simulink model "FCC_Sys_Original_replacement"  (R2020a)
settings: Solver=FixedStepDiscrete  StartTime=0.0  StopTime=10.0  FixedStep=0.001  RelTol=1e-3  EnableMultiTasking=on
model workspace (MAT data in the model file):
  Ts : Simulink.Parameter (value not decoded)
  carriedVarFromRefMdlDV_0_Ts = 0.01
symbols that are objects in the model workspace (value not decoded): Ts
undefined symbols (not defined in the file or in its folder): ActuatorLoop, AHRS_voter, DiscIntNeverNeededParam, FCC, Heli_inner_loop, Heli_outer_loop, Kd, Ki, Kp, Normal
libraries: simulink x10, HeliLibrary x3

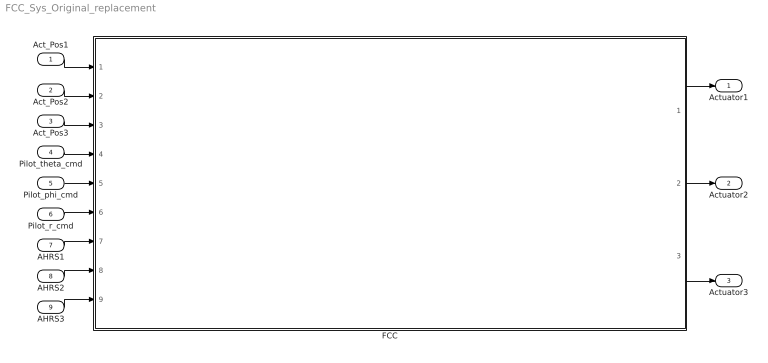
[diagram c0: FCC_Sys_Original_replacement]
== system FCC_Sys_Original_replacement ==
  Act_Pos1 : Inport  OutMin=-32768  OutMax=32767  OutDataTypeStr=int16  PortDimensions=1  SampleTime=0.001
  Act_Pos2 : Inport  Port=2  OutMin=-32768  OutMax=32767  OutDataTypeStr=int16  PortDimensions=1  SampleTime=0.001
  Act_Pos3 : Inport  Port=3  OutMin=-32768  OutMax=32767  OutDataTypeStr=int16  PortDimensions=1  SampleTime=0.001
  Pilot_theta_cmd : Inport  Port=4  OutMin=-32768  OutMax=32767  OutDataTypeStr=int16  PortDimensions=1  SampleTime=0.01
  Pilot_phi_cmd : Inport  Port=5  OutMin=-32768  OutMax=32767  OutDataTypeStr=int16  PortDimensions=1  SampleTime=0.01
  Pilot_r_cmd : Inport  Port=6  OutMin=-32768  OutMax=32767  OutDataTypeStr=int16  PortDimensions=1  SampleTime=0.01
  AHRS1 : Inport  Port=7  OutDataTypeStr=Bus: AHRS_Bus  PortDimensions=1  SampleTime=0.01
  AHRS2 : Inport  Port=8  OutDataTypeStr=Bus: AHRS_Bus  PortDimensions=1  SampleTime=0.01
  AHRS3 : Inport  Port=9  OutDataTypeStr=Bus: AHRS_Bus  PortDimensions=1  SampleTime=0.01
  FCC : Subsystem  TreatAsAtomicUnit=on  mask(Sldv ModelReference(Model name:FCC) Replacement){ModelName=FCC, ParameterArgumentNames=, ParameterArgumentValuesAsString=, SimulationMode=Normal}
      mask help: Replacement for the Model Reference block that references the model FCC. If Model arguments are specified on the Model Reference block, then they will appear in the mask parameters.
  Actuator1 : Outport  VectorParamsAs1DForOutWhenUnconnected=off
  Actuator2 : Outport  Port=2  VectorParamsAs1DForOutWhenUnconnected=off
  Actuator3 : Outport  Port=3  VectorParamsAs1DForOutWhenUnconnected=off
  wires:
  Act_Pos1/1 -> FCC/1(Act_Pos1)
  Act_Pos2/1 -> FCC/2(Act_Pos2)
  Act_Pos3/1 -> FCC/3(Act_Pos3)
  Pilot_theta_cmd/1 -> FCC/4(Pilot_theta_cmd)
  Pilot_phi_cmd/1 -> FCC/5(Pilot_phi_cmd)
  Pilot_r_cmd/1 -> FCC/6(Pilot_r_cmd)
  AHRS1/1 -> FCC/7(AHRS1)
  AHRS2/1 -> FCC/8(AHRS2)
  AHRS3/1 -> FCC/9(AHRS3)
  FCC/1(Actuator1) -> Actuator1/1
  FCC/2(Actuator2) -> Actuator2/1
  FCC/3(Actuator3) -> Actuator3/1

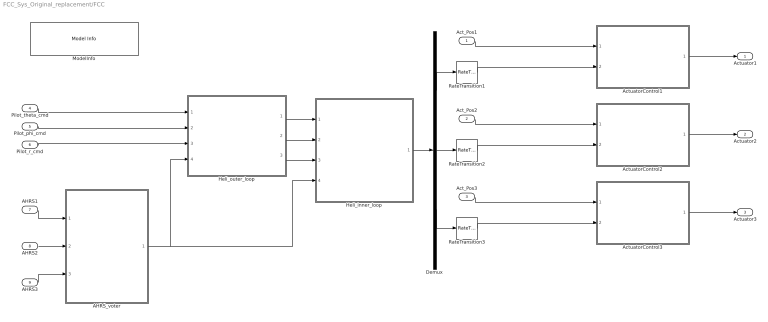
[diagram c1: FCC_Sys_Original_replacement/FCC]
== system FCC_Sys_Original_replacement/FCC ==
  Act_Pos1 : Inport  OutMin=-32768  OutMax=32767  OutDataTypeStr=int16  PortDimensions=1  SampleTime=[0.001,0]
  Act_Pos2 : Inport  Port=2  OutMin=-32768  OutMax=32767  OutDataTypeStr=int16  PortDimensions=1  SampleTime=[0.001,0]
  Act_Pos3 : Inport  Port=3  OutMin=-32768  OutMax=32767  OutDataTypeStr=int16  PortDimensions=1  SampleTime=[0.001,0]
  Pilot_theta_cmd : Inport  Port=4  OutMin=-32768  OutMax=32767  OutDataTypeStr=int16  PortDimensions=1  SampleTime=[0.01,0]
  Pilot_phi_cmd : Inport  Port=5  OutMin=-32768  OutMax=32767  OutDataTypeStr=int16  PortDimensions=1  SampleTime=[0.01,0]
  Pilot_r_cmd : Inport  Port=6  OutMin=-32768  OutMax=32767  OutDataTypeStr=int16  PortDimensions=1  SampleTime=[0.01,0]
  AHRS1 : Inport  Port=7  OutDataTypeStr=Bus: AHRS_Bus  PortDimensions=1  SampleTime=[0.01,0]
  AHRS2 : Inport  Port=8  OutDataTypeStr=Bus: AHRS_Bus  PortDimensions=1  SampleTime=[0.01,0]
  AHRS3 : Inport  Port=9  OutDataTypeStr=Bus: AHRS_Bus  PortDimensions=1  SampleTime=[0.01,0]
  AHRS_voter : Subsystem  TreatAsAtomicUnit=on  mask(Sldv ModelReference(Model name:AHRS_voter) Replacement){ModelName=AHRS_voter, ParameterArgumentNames=, ParameterArgumentValuesAsString=, SimulationMode=Normal}
      mask help: Replacement for the Model Reference block that references the model AHRS_voter. If Model arguments are specified on the Model Reference block, then they will appear in the mask parameters.
  ActuatorControl1 : Subsystem  TreatAsAtomicUnit=on  mask(Sldv ModelReference(Model name:ActuatorLoop) Replacement){Kd=double(0.00272), Ki=double(2.73), Kp=double(0.339), ModelName=ActuatorLoop, ParameterArgumentNames=Kd,Ki,Kp, ParameterArgumentValuesAsString=0.00272,2.73,0.339, SimulationMode=Normal}
      mask help: Replacement for the Model Reference block that references the model ActuatorLoop. If Model arguments are specified on the Model Reference block, then they will appear in the mask parameters.
  ActuatorControl2 : Subsystem  TreatAsAtomicUnit=on  mask(Sldv ModelReference(Model name:ActuatorLoop) Replacement){Kd=double(0.00272), Ki=double(2.73), Kp=double(0.339), ModelName=ActuatorLoop, ParameterArgumentNames=Kd,Ki,Kp, ParameterArgumentValuesAsString=0.00272,2.73,0.339, SimulationMode=Normal}
      mask help: Replacement for the Model Reference block that references the model ActuatorLoop. If Model arguments are specified on the Model Reference block, then they will appear in the mask parameters.
  ActuatorControl3 : Subsystem  TreatAsAtomicUnit=on  mask(Sldv ModelReference(Model name:ActuatorLoop) Replacement){Kd=double(0.00272), Ki=double(2.73), Kp=double(0.339), ModelName=ActuatorLoop, ParameterArgumentNames=Kd,Ki,Kp, ParameterArgumentValuesAsString=0.00272,2.73,0.339, SimulationMode=Normal}
      mask help: Replacement for the Model Reference block that references the model ActuatorLoop. If Model arguments are specified on the Model Reference block, then they will appear in the mask parameters.
  Demux : Demux  Outputs=3
  Heli_inner_loop : Subsystem  TreatAsAtomicUnit=on  mask(Sldv ModelReference(Model name:Heli_inner_loop) Replacement){ModelName=Heli_inner_loop, ParameterArgumentNames=, ParameterArgumentValuesAsString=, SimulationMode=Normal}
      mask help: Replacement for the Model Reference block that references the model Heli_inner_loop. If Model arguments are specified on the Model Reference block, then they will appear in the mask parameters.
  Heli_outer_loop : Subsystem  TreatAsAtomicUnit=on  mask(Sldv ModelReference(Model name:Heli_outer_loop) Replacement){Ts=carriedVarFromRefMdlDV_0_Ts, ModelName=Heli_outer_loop, ParameterArgumentNames=, ParameterArgumentValuesAsString=, SimulationMode=Normal}
      mask help: Replacement for the Model Reference block that references the model Heli_outer_loop. If Model arguments are specified on the Model Reference block, then they will appear in the mask parameters.
  ModelInfo : simulink/Model-Wide Utilities/Model Info  Frame=on  DisplayStringWithTags=|  HorizontalTextAlignment=Center  LeftAlignmentValue=0.5
      | Model Name: %<ModelName>
      | Model Version: %<ModelVersion>
      | Last Modified: %<LastModificationDate>
      | 
      | Copyright 2016 The MathWorks, Inc.
  RateTransition1 : RateTransition  OutPortSampleTime=0.001
  RateTransition2 : RateTransition  OutPortSampleTime=0.001
  RateTransition3 : RateTransition  OutPortSampleTime=0.001
  Actuator1 : Outport  OutDataTypeStr=int16  PortDimensions=1  SampleTime=[0.001,0]  VectorParamsAs1DForOutWhenUnconnected=off
  Actuator2 : Outport  Port=2  OutDataTypeStr=int16  PortDimensions=1  SampleTime=[0.001,0]  VectorParamsAs1DForOutWhenUnconnected=off
  Actuator3 : Outport  Port=3  OutDataTypeStr=int16  PortDimensions=1  SampleTime=[0.001,0]  VectorParamsAs1DForOutWhenUnconnected=off
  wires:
  AHRS_voter/1(voted_fb) -> Heli_inner_loop/4(voted_fb), Heli_outer_loop/4(voted_fb)
  ActuatorControl3/1(ActuatorCommand) -> Actuator3/1
  ActuatorControl2/1(ActuatorCommand) -> Actuator2/1
  ActuatorControl1/1(ActuatorCommand) -> Actuator1/1
  Act_Pos3/1 -> ActuatorControl3/1(PositionFeedback)
  Act_Pos2/1 -> ActuatorControl2/1(PositionFeedback)
  Act_Pos1/1 -> ActuatorControl1/1(PositionFeedback)
  Pilot_r_cmd/1 -> Heli_outer_loop/3(Pilot_r_cmd)
  Pilot_phi_cmd/1 -> Heli_outer_loop/2(Pilot_phi_cmd)
  Pilot_theta_cmd/1 -> Heli_outer_loop/1(Pilot_theta_cmd)
  AHRS1/1 -> AHRS_voter/1(AHRS1)
  Heli_outer_loop/3(r_cmd) -> Heli_inner_loop/3(r_cmd)
  Heli_outer_loop/2(phi_cmd) -> Heli_inner_loop/2(phi_cmd)
  Heli_outer_loop/1(theta_cmd) -> Heli_inner_loop/1(theta_cmd)
  Heli_inner_loop/1(actuator_commands) -> Demux/1
  Demux/3 -> RateTransition3/1
  Demux/2 -> RateTransition2/1
  Demux/1 -> RateTransition1/1
  AHRS3/1 -> AHRS_voter/3(AHRS3)
  AHRS2/1 -> AHRS_voter/2(AHRS2)
  RateTransition3/1 -> ActuatorControl3/2(PositionCommand)
  RateTransition2/1 -> ActuatorControl2/2(PositionCommand)
  RateTransition1/1 -> ActuatorControl1/2(PositionCommand)

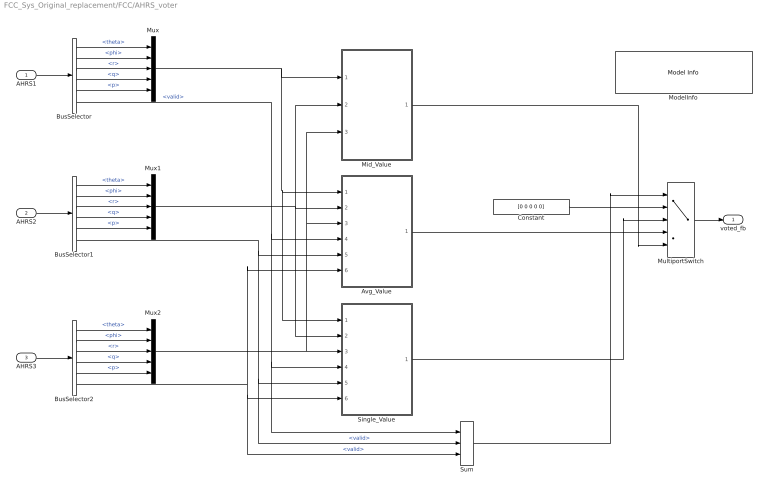
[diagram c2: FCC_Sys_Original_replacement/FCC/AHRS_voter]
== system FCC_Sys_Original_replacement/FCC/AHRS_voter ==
  AHRS1 : Inport  OutDataTypeStr=Bus: AHRS_Bus  PortDimensions=1  SampleTime=[0.01,0]
  AHRS2 : Inport  Port=2  OutDataTypeStr=Bus: AHRS_Bus  PortDimensions=1  SampleTime=[0.01,0]
  AHRS3 : Inport  Port=3  OutDataTypeStr=Bus: AHRS_Bus  PortDimensions=1  SampleTime=[0.01,0]
  Avg_Value : Subsystem  TreatAsAtomicUnit=on  RTWFcnName=Avg_Value
  BusSelector : BusSelector  OutputSignals=theta,phi,r,q,p,valid
  BusSelector1 : BusSelector  OutputSignals=theta,phi,r,q,p,valid
  BusSelector2 : BusSelector  OutputSignals=theta,phi,r,q,p,valid
  Constant : Constant  Value=[0 0 0 0 0]
  Mid_Value : Subsystem  TreatAsAtomicUnit=on  RTWFcnName=Mid_Value
  ModelInfo : simulink/Model-Wide Utilities/Model Info  Frame=on  DisplayStringWithTags=|  HorizontalTextAlignment=Center  LeftAlignmentValue=0.5
      | Model Name: %<ModelName>
      | Model Version: %<ModelVersion>
      | Last Modified: %<LastModificationDate>
      | 
      | Copyright 2016 The MathWorks, Inc.
  MultiportSwitch : MultiPortSwitch  DataPortOrder=Zero-based contiguous  Inputs=4  DiagnosticForDefault=None  zeroidx=on
  Mux : Mux  Inputs=5
  Mux1 : Mux  Inputs=5
  Mux2 : Mux  Inputs=5
  Single_Value : Subsystem  TreatAsAtomicUnit=on  RTWFcnName=Single_Value
  Sum : Sum  Inputs=+++  OutDataTypeStr=uint32
  voted_fb : Outport  OutDataTypeStr=double  PortDimensions=5  SampleTime=[0.01,0]  VectorParamsAs1DForOutWhenUnconnected=off
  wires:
  BusSelector2/6 -> Single_Value/6(AHRS3_Valid), Sum/3, Avg_Value/6(AHRS3_Valid)  "<valid>"
  BusSelector2/5 -> Mux2/5  "<p>"
  BusSelector2/4 -> Mux2/4  "<q>"
  BusSelector2/3 -> Mux2/3  "<r>"
  BusSelector2/2 -> Mux2/2  "<phi>"
  BusSelector2/1 -> Mux2/1  "<theta>"
  AHRS3/1 -> BusSelector2/1
  Mux2/1 -> Mid_Value/3(AHRS3), Avg_Value/3(AHRS3), Single_Value/3(AHRS3)
  BusSelector1/6 -> Avg_Value/5(AHRS2_Valid), Sum/2, Single_Value/5(AHRS2_Valid)  "<valid>"
  Mux1/1 -> Single_Value/2(AHRS2), Mid_Value/2(AHRS2), Avg_Value/2(AHRS2)
  AHRS2/1 -> BusSelector1/1
  BusSelector1/1 -> Mux1/1  "<theta>"
  BusSelector1/2 -> Mux1/2  "<phi>"
  BusSelector1/3 -> Mux1/3  "<r>"
  BusSelector1/4 -> Mux1/4  "<q>"
  BusSelector1/5 -> Mux1/5  "<p>"
  Mux/1 -> Single_Value/1(AHRS1), Avg_Value/1(AHRS1), Mid_Value/1(AHRS1)
  BusSelector/5 -> Mux/5  "<p>"
  BusSelector/4 -> Mux/4  "<q>"
  BusSelector/3 -> Mux/3  "<r>"
  BusSelector/2 -> Mux/2  "<phi>"
  BusSelector/1 -> Mux/1  "<theta>"
  BusSelector/6 -> Single_Value/4(AHRS1_Valid), Sum/1, Avg_Value/4(AHRS1_Valid)  "<valid>"
  AHRS1/1 -> BusSelector/1
  Constant/1 -> MultiportSwitch/2
  Single_Value/1(Single_Value) -> MultiportSwitch/3
  Avg_Value/1(Avg_Value) -> MultiportSwitch/4
  Mid_Value/1(Mid_Value) -> MultiportSwitch/5
  Sum/1 -> MultiportSwitch/1
  MultiportSwitch/1 -> voted_fb/1

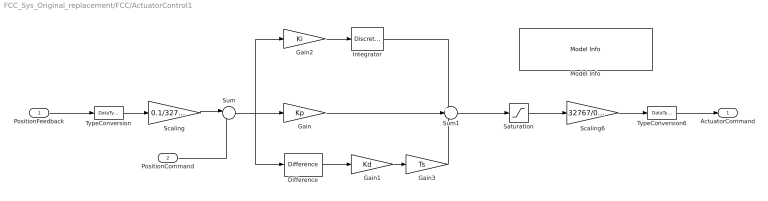
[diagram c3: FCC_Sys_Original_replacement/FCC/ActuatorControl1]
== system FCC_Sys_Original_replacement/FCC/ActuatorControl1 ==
  PositionFeedback : Inport  OutMin=-32768  OutMax=32767  OutDataTypeStr=int16  PortDimensions=1  SampleTime=[0.001,0]
  PositionCommand : Inport  Port=2  OutMin=-0.1  OutMax=0.1  OutDataTypeStr=double  PortDimensions=1  SampleTime=[0.001,0]
  Difference : simulink/Discrete/Difference  ICPrevInput=0.0  OutMin=[]  OutMax=[]  OutDataType=fixdt(1, 16)  OutScaling=2^-10  DoSatur=off
  Gain : Gain  Gain=Kp
  Gain1 : Gain  Gain=Kd
  Gain2 : Gain  Gain=Ki
  Gain3 : Gain  Gain=Ts
  Integrator : DiscreteIntegrator  SampleTime=-1  LimitOutput=on  UpperSaturationLimit=0.1  LowerSaturationLimit=-0.1  ICPrevOutput=DiscIntNeverNeededParam  ICPrevScaledInput=DiscIntNeverNeededParam
  Model Info : simulink/Model-Wide Utilities/Model Info  Frame=on  DisplayStringWithTags=|  HorizontalTextAlignment=Center  LeftAlignmentValue=0.5
      | Model Name: %<ModelName>
      | Model Version: %<ModelVersion>
      | Last Modified: %<LastModificationDate>
      | 
      | Copyright 2016 The MathWorks, Inc.
  Saturation : Saturate  UpperLimit=0.3  LowerLimit=-0.3
  Scaling : Gain  Gain=0.1/32767
  Scaling6 : Gain  Gain=32767/0.3  SaturateOnIntegerOverflow=on
  Sum : Sum  Inputs=|-+
  Sum1 : Sum  Inputs=++-
  TypeConversion : DataTypeConversion  OutDataTypeStr=double
  TypeConversion6 : DataTypeConversion  OutDataTypeStr=int16
  ActuatorCommand : Outport  OutDataTypeStr=int16  PortDimensions=1  SampleTime=[0.001,0]  VectorParamsAs1DForOutWhenUnconnected=off
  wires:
  Gain3/1 -> Sum1/3
  TypeConversion6/1 -> ActuatorCommand/1
  Saturation/1 -> Scaling6/1
  Scaling6/1 -> TypeConversion6/1
  Scaling/1 -> Sum/1
  TypeConversion/1 -> Scaling/1
  PositionFeedback/1 -> TypeConversion/1
  Gain2/1 -> Integrator/1
  Gain1/1 -> Gain3/1
  Difference/1 -> Gain1/1
  Integrator/1 -> Sum1/1
  Sum1/1 -> Saturation/1
  Gain/1 -> Sum1/2
  Sum/1 -> Difference/1, Gain2/1, Gain/1
  PositionCommand/1 -> Sum/2

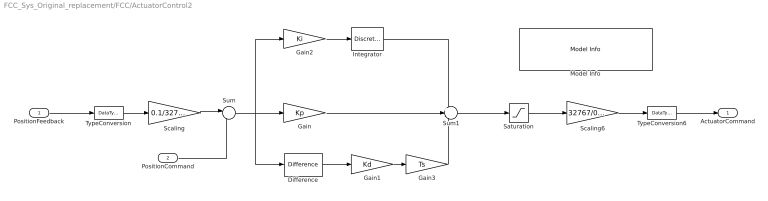
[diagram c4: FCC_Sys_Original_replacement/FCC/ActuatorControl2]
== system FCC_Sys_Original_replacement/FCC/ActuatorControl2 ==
  PositionFeedback : Inport  OutMin=-32768  OutMax=32767  OutDataTypeStr=int16  PortDimensions=1  SampleTime=[0.001,0]
  PositionCommand : Inport  Port=2  OutMin=-0.1  OutMax=0.1  OutDataTypeStr=double  PortDimensions=1  SampleTime=[0.001,0]
  Difference : simulink/Discrete/Difference  ICPrevInput=0.0  OutMin=[]  OutMax=[]  OutDataType=fixdt(1, 16)  OutScaling=2^-10  DoSatur=off
  Gain : Gain  Gain=Kp
  Gain1 : Gain  Gain=Kd
  Gain2 : Gain  Gain=Ki
  Gain3 : Gain  Gain=Ts
  Integrator : DiscreteIntegrator  SampleTime=-1  LimitOutput=on  UpperSaturationLimit=0.1  LowerSaturationLimit=-0.1  ICPrevOutput=DiscIntNeverNeededParam  ICPrevScaledInput=DiscIntNeverNeededParam
  Model Info : simulink/Model-Wide Utilities/Model Info  Frame=on  DisplayStringWithTags=|  HorizontalTextAlignment=Center  LeftAlignmentValue=0.5
      | Model Name: %<ModelName>
      | Model Version: %<ModelVersion>
      | Last Modified: %<LastModificationDate>
      | 
      | Copyright 2016 The MathWorks, Inc.
  Saturation : Saturate  UpperLimit=0.3  LowerLimit=-0.3
  Scaling : Gain  Gain=0.1/32767
  Scaling6 : Gain  Gain=32767/0.3  SaturateOnIntegerOverflow=on
  Sum : Sum  Inputs=|-+
  Sum1 : Sum  Inputs=++-
  TypeConversion : DataTypeConversion  OutDataTypeStr=double
  TypeConversion6 : DataTypeConversion  OutDataTypeStr=int16
  ActuatorCommand : Outport  OutDataTypeStr=int16  PortDimensions=1  SampleTime=[0.001,0]  VectorParamsAs1DForOutWhenUnconnected=off
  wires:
  Gain3/1 -> Sum1/3
  TypeConversion6/1 -> ActuatorCommand/1
  Saturation/1 -> Scaling6/1
  Scaling6/1 -> TypeConversion6/1
  Scaling/1 -> Sum/1
  TypeConversion/1 -> Scaling/1
  PositionFeedback/1 -> TypeConversion/1
  Gain2/1 -> Integrator/1
  Gain1/1 -> Gain3/1
  Difference/1 -> Gain1/1
  Integrator/1 -> Sum1/1
  Sum1/1 -> Saturation/1
  Gain/1 -> Sum1/2
  Sum/1 -> Difference/1, Gain2/1, Gain/1
  PositionCommand/1 -> Sum/2

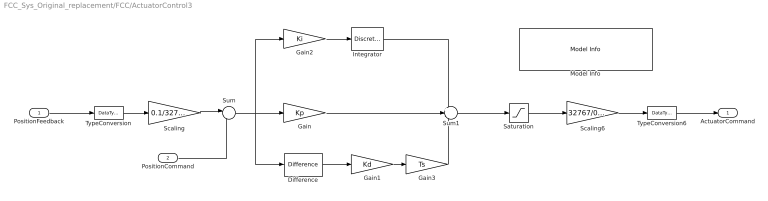
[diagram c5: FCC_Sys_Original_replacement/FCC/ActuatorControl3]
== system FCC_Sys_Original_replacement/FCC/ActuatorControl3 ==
  PositionFeedback : Inport  OutMin=-32768  OutMax=32767  OutDataTypeStr=int16  PortDimensions=1  SampleTime=[0.001,0]
  PositionCommand : Inport  Port=2  OutMin=-0.1  OutMax=0.1  OutDataTypeStr=double  PortDimensions=1  SampleTime=[0.001,0]
  Difference : simulink/Discrete/Difference  ICPrevInput=0.0  OutMin=[]  OutMax=[]  OutDataType=fixdt(1, 16)  OutScaling=2^-10  DoSatur=off
  Gain : Gain  Gain=Kp
  Gain1 : Gain  Gain=Kd
  Gain2 : Gain  Gain=Ki
  Gain3 : Gain  Gain=Ts
  Integrator : DiscreteIntegrator  SampleTime=-1  LimitOutput=on  UpperSaturationLimit=0.1  LowerSaturationLimit=-0.1  ICPrevOutput=DiscIntNeverNeededParam  ICPrevScaledInput=DiscIntNeverNeededParam
  Model Info : simulink/Model-Wide Utilities/Model Info  Frame=on  DisplayStringWithTags=|  HorizontalTextAlignment=Center  LeftAlignmentValue=0.5
      | Model Name: %<ModelName>
      | Model Version: %<ModelVersion>
      | Last Modified: %<LastModificationDate>
      | 
      | Copyright 2016 The MathWorks, Inc.
  Saturation : Saturate  UpperLimit=0.3  LowerLimit=-0.3
  Scaling : Gain  Gain=0.1/32767
  Scaling6 : Gain  Gain=32767/0.3  SaturateOnIntegerOverflow=on
  Sum : Sum  Inputs=|-+
  Sum1 : Sum  Inputs=++-
  TypeConversion : DataTypeConversion  OutDataTypeStr=double
  TypeConversion6 : DataTypeConversion  OutDataTypeStr=int16
  ActuatorCommand : Outport  OutDataTypeStr=int16  PortDimensions=1  SampleTime=[0.001,0]  VectorParamsAs1DForOutWhenUnconnected=off
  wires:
  Gain3/1 -> Sum1/3
  TypeConversion6/1 -> ActuatorCommand/1
  Saturation/1 -> Scaling6/1
  Scaling6/1 -> TypeConversion6/1
  Scaling/1 -> Sum/1
  TypeConversion/1 -> Scaling/1
  PositionFeedback/1 -> TypeConversion/1
  Gain2/1 -> Integrator/1
  Gain1/1 -> Gain3/1
  Difference/1 -> Gain1/1
  Integrator/1 -> Sum1/1
  Sum1/1 -> Saturation/1
  Gain/1 -> Sum1/2
  Sum/1 -> Difference/1, Gain2/1, Gain/1
  PositionCommand/1 -> Sum/2

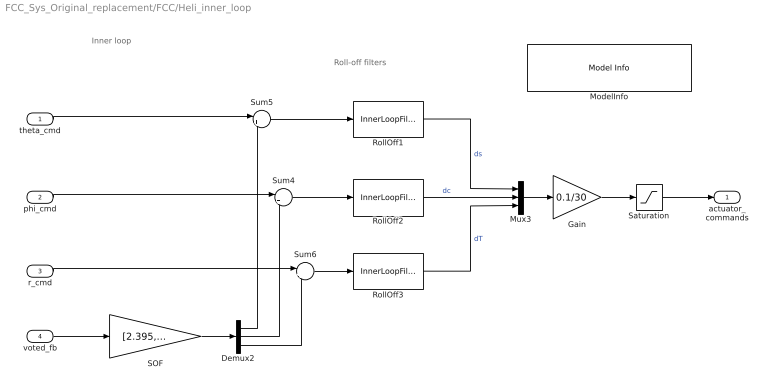
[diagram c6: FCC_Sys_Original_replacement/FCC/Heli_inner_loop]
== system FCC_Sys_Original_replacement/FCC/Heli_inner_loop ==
  note: Inner loop
  note: Roll-off filters
  theta_cmd : Inport  OutMin=-30  OutMax=30  OutDataTypeStr=double  PortDimensions=1  SampleTime=[0.01,0]
  phi_cmd : Inport  Port=2  OutMin=-30  OutMax=30  OutDataTypeStr=double  PortDimensions=1  SampleTime=[0.01,0]
  r_cmd : Inport  Port=3  OutMin=-30  OutMax=30  OutDataTypeStr=double  PortDimensions=1  SampleTime=[0.01,0]
  voted_fb : Inport  Port=4  OutMin=-180  OutMax=180  OutDataTypeStr=double  PortDimensions=5  SampleTime=[0.01,0]
  Demux2 : Demux  Outputs=3
  Gain : Gain  Gain=0.1/30
  ModelInfo : simulink/Model-Wide Utilities/Model Info  Frame=on  DisplayStringWithTags=|  HorizontalTextAlignment=Center  LeftAlignmentValue=0.5
      | Model Name: %<ModelName>
      | Model Version: %<ModelVersion>
      | Last Modified: %<LastModificationDate>
      | 
      | Copyright 2016 The MathWorks, Inc.
  Mux3 : Mux  Inputs=3
  RollOff1 : HeliLibrary/InnerLoopFilter  Tag=FilterWizardSubSystem  SystemSampleTime=-1  Latency=0  AutoFrameSizeCalculation=off
  RollOff2 : HeliLibrary/InnerLoopFilter  Tag=FilterWizardSubSystem  SystemSampleTime=-1  Latency=0  AutoFrameSizeCalculation=off
  RollOff3 : HeliLibrary/InnerLoopFilter  Tag=FilterWizardSubSystem  SystemSampleTime=-1  Latency=0  AutoFrameSizeCalculation=off
  SOF : Gain  Gain=[2.395, -0.3609, -0.002145, 0.8087, -0.0205; -0.1427, -1.115, 0.04573, -0.04318, -0.1007; -0.02792, -0.02229, -2.025, -0.06152, 0.03151;]  Multiplication=Matrix(K*u) (u vector)
  Saturation : Saturate  UpperLimit=0.1  LowerLimit=-0.1
  Sum4 : Sum  Inputs=|+-
  Sum5 : Sum  Inputs=|+-
  Sum6 : Sum  Inputs=|+-
  actuator_commands : Outport  OutDataTypeStr=double  PortDimensions=3  SampleTime=[0.01,0]  VectorParamsAs1DForOutWhenUnconnected=off
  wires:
  Saturation/1 -> actuator_commands/1
  Gain/1 -> Saturation/1
  voted_fb/1 -> SOF/1
  Demux2/3 -> Sum6/2
  Demux2/2 -> Sum4/2
  Demux2/1 -> Sum5/2
  Sum6/1 -> RollOff3/1
  r_cmd/1 -> Sum6/1
  phi_cmd/1 -> Sum4/1
  SOF/1 -> Demux2/1
  Sum5/1 -> RollOff1/1
  theta_cmd/1 -> Sum5/1
  RollOff1/1 -> Mux3/1  "ds"
  RollOff2/1 -> Mux3/2  "dc"
  RollOff3/1 -> Mux3/3  "dT"
  Sum4/1 -> RollOff2/1
  Mux3/1 -> Gain/1

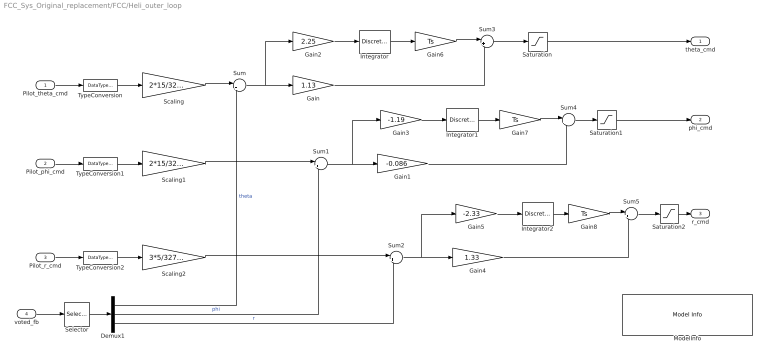
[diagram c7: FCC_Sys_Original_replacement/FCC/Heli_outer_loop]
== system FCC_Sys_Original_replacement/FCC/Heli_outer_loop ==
  Pilot_theta_cmd : Inport  OutMin=-32768  OutMax=32767  OutDataTypeStr=int16  PortDimensions=1  SampleTime=[0.01,0]
  Pilot_phi_cmd : Inport  Port=2  OutMin=-32768  OutMax=32767  OutDataTypeStr=int16  PortDimensions=1  SampleTime=[0.01,0]
  Pilot_r_cmd : Inport  Port=3  OutMin=-32768  OutMax=32767  OutDataTypeStr=int16  PortDimensions=1  SampleTime=[0.01,0]
  voted_fb : Inport  Port=4  OutMin=-180  OutMax=180  OutDataTypeStr=double  PortDimensions=5  SampleTime=[0.01,0]
  Demux1 : Demux  Outputs=3
  Gain : Gain  Gain=1.13
  Gain1 : Gain  Gain=-0.086
  Gain2 : Gain  Gain=2.25
  Gain3 : Gain  Gain=-1.19
  Gain4 : Gain  Gain=1.33
  Gain5 : Gain  Gain=-2.33
  Gain6 : Gain  Gain=Ts
  Gain7 : Gain  Gain=Ts
  Gain8 : Gain  Gain=Ts
  Integrator : DiscreteIntegrator  IntegratorMethod=Accumulation: Forward Euler  SampleTime=-1  LimitOutput=on  UpperSaturationLimit=10  LowerSaturationLimit=-10  ICPrevOutput=DiscIntNeverNeededParam  ICPrevScaledInput=DiscIntNeverNeededParam
  Integrator1 : DiscreteIntegrator  IntegratorMethod=Accumulation: Forward Euler  SampleTime=-1  LimitOutput=on  UpperSaturationLimit=10  LowerSaturationLimit=-10  ICPrevOutput=DiscIntNeverNeededParam  ICPrevScaledInput=DiscIntNeverNeededParam
  Integrator2 : DiscreteIntegrator  IntegratorMethod=Accumulation: Forward Euler  SampleTime=-1  LimitOutput=on  UpperSaturationLimit=10  LowerSaturationLimit=-10  ICPrevOutput=DiscIntNeverNeededParam  ICPrevScaledInput=DiscIntNeverNeededParam
  ModelInfo : simulink/Model-Wide Utilities/Model Info  Frame=on  DisplayStringWithTags=|  HorizontalTextAlignment=Center  LeftAlignmentValue=0.5
      | Model Name: %<ModelName>
      | Model Version: %<ModelVersion>
      | Last Modified: %<LastModificationDate>
      | 
      | Copyright 2016 The MathWorks, Inc.
  Saturation : Saturate  UpperLimit=30  LowerLimit=-30
  Saturation1 : Saturate  UpperLimit=30  LowerLimit=-30
  Saturation2 : Saturate  UpperLimit=30  LowerLimit=-30
  Scaling : Gain  Gain=2*15/32767
  Scaling1 : Gain  Gain=2*15/32767
  Scaling2 : Gain  Gain=3*5/32767
  Selector : Selector  InputPortWidth=5  IndexOptions=Index vector (dialog)  Indices=[1 2 3]  OutputSizes=1
  Sum : Sum  Inputs=|+-  InputSameDT=on
  Sum1 : Sum  Inputs=|+-  InputSameDT=on
  Sum2 : Sum  Inputs=|+-  InputSameDT=on
  Sum3 : Sum  Inputs=|++
  Sum4 : Sum  Inputs=|++
  Sum5 : Sum  Inputs=|++
  TypeConversion : DataTypeConversion  OutDataTypeStr=double
  TypeConversion1 : DataTypeConversion  OutDataTypeStr=double
  TypeConversion2 : DataTypeConversion  OutDataTypeStr=double
  theta_cmd : Outport  OutDataTypeStr=double  PortDimensions=1  SampleTime=[0.01,0]  VectorParamsAs1DForOutWhenUnconnected=off
  phi_cmd : Outport  Port=2  OutDataTypeStr=double  PortDimensions=1  SampleTime=[0.01,0]  VectorParamsAs1DForOutWhenUnconnected=off
  r_cmd : Outport  Port=3  OutDataTypeStr=double  PortDimensions=1  SampleTime=[0.01,0]  VectorParamsAs1DForOutWhenUnconnected=off
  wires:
  Gain8/1 -> Sum5/1
  Gain7/1 -> Sum4/1
  Gain6/1 -> Sum3/1
  Scaling2/1 -> Sum2/1
  Pilot_r_cmd/1 -> TypeConversion2/1
  Scaling1/1 -> Sum1/1
  Pilot_phi_cmd/1 -> TypeConversion1/1
  Scaling/1 -> Sum/1
  Pilot_theta_cmd/1 -> TypeConversion/1
  TypeConversion/1 -> Scaling/1
  TypeConversion1/1 -> Scaling1/1
  TypeConversion2/1 -> Scaling2/1
  Saturation2/1 -> r_cmd/1
  Sum2/1 -> Gain5/1, Gain4/1
  Gain5/1 -> Integrator2/1
  Integrator2/1 -> Gain8/1
  Sum5/1 -> Saturation2/1
  Gain4/1 -> Sum5/2
  Saturation1/1 -> phi_cmd/1
  Gain3/1 -> Integrator1/1
  Integrator1/1 -> Gain7/1
  Sum4/1 -> Saturation1/1
  Gain1/1 -> Sum4/2
  Sum1/1 -> Gain3/1, Gain1/1
  Saturation/1 -> theta_cmd/1
  Gain2/1 -> Integrator/1
  Integrator/1 -> Gain6/1
  Sum3/1 -> Saturation/1
  Gain/1 -> Sum3/2
  Sum/1 -> Gain/1, Gain2/1
  voted_fb/1 -> Selector/1
  Demux1/3 -> Sum2/2  "r"
  Demux1/2 -> Sum1/2  "phi"
  Demux1/1 -> Sum/2  "theta"
  Selector/1 -> Demux1/1

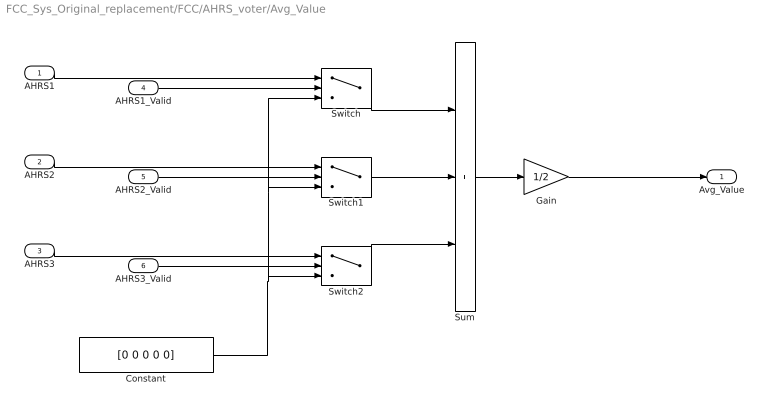
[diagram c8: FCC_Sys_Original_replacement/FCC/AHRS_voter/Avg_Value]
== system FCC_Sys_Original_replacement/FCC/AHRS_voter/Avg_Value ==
  AHRS1 : Inport
  AHRS2 : Inport  Port=2
  AHRS3 : Inport  Port=3
  AHRS1_Valid : Inport  Port=4  OutDataTypeStr=boolean  PortDimensions=1
  AHRS2_Valid : Inport  Port=5  OutDataTypeStr=boolean  PortDimensions=1
  AHRS3_Valid : Inport  Port=6  OutDataTypeStr=boolean  PortDimensions=1
  Constant : Constant  Value=[0 0 0 0 0]
  Gain : Gain  Gain=1/2
  Sum : Sum  Inputs=+++
  Switch : Switch  Criteria=u2 ~= 0
  Switch1 : Switch  Criteria=u2 ~= 0
  Switch2 : Switch  Criteria=u2 ~= 0
  Avg_Value : Outport  VectorParamsAs1DForOutWhenUnconnected=off
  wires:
  Gain/1 -> Avg_Value/1
  Sum/1 -> Gain/1
  AHRS1_Valid/1 -> Switch/2
  AHRS1/1 -> Switch/1
  Switch/1 -> Sum/1
  Switch1/1 -> Sum/2
  Switch2/1 -> Sum/3
  AHRS2_Valid/1 -> Switch1/2
  AHRS3_Valid/1 -> Switch2/2
  AHRS2/1 -> Switch1/1
  AHRS3/1 -> Switch2/1
  Constant/1 -> Switch/3, Switch1/3, Switch2/3

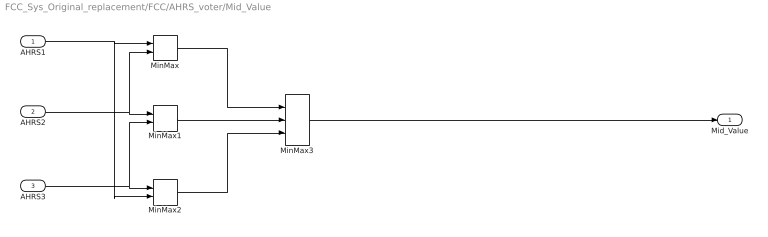
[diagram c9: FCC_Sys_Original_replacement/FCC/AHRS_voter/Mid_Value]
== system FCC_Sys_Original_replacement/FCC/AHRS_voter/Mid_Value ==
  AHRS1 : Inport
  AHRS2 : Inport  Port=2
  AHRS3 : Inport  Port=3
  MinMax : MinMax  Inputs=2
  MinMax1 : MinMax  Inputs=2
  MinMax2 : MinMax  Inputs=2
  MinMax3 : MinMax  Function=max  Inputs=3
  Mid_Value : Outport  VectorParamsAs1DForOutWhenUnconnected=off
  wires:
  AHRS1/1 -> MinMax2/2, MinMax/1
  AHRS3/1 -> MinMax1/2, MinMax2/1
  AHRS2/1 -> MinMax/2, MinMax1/1
  MinMax1/1 -> MinMax3/2
  MinMax/1 -> MinMax3/1
  MinMax2/1 -> MinMax3/3
  MinMax3/1 -> Mid_Value/1

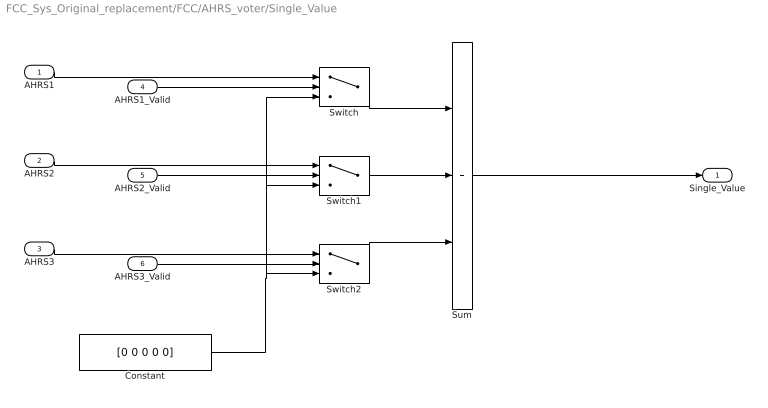
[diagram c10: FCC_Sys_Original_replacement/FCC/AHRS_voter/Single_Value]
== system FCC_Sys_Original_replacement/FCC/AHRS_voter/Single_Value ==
  AHRS1 : Inport
  AHRS2 : Inport  Port=2
  AHRS3 : Inport  Port=3
  AHRS1_Valid : Inport  Port=4  OutDataTypeStr=boolean  PortDimensions=1
  AHRS2_Valid : Inport  Port=5  OutDataTypeStr=boolean  PortDimensions=1
  AHRS3_Valid : Inport  Port=6  OutDataTypeStr=boolean  PortDimensions=1
  Constant : Constant  Value=[0 0 0 0 0]
  Sum : Sum  Inputs=+++
  Switch : Switch  Criteria=u2 ~= 0
  Switch1 : Switch  Criteria=u2 ~= 0
  Switch2 : Switch  Criteria=u2 ~= 0
  Single_Value : Outport  VectorParamsAs1DForOutWhenUnconnected=off
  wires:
  Constant/1 -> Switch2/3, Switch1/3, Switch/3
  AHRS3/1 -> Switch2/1
  AHRS2/1 -> Switch1/1
  AHRS3_Valid/1 -> Switch2/2
  AHRS2_Valid/1 -> Switch1/2
  Switch2/1 -> Sum/3
  Switch1/1 -> Sum/2
  Switch/1 -> Sum/1
  AHRS1/1 -> Switch/1
  AHRS1_Valid/1 -> Switch/2
  Sum/1 -> Single_Value/1
